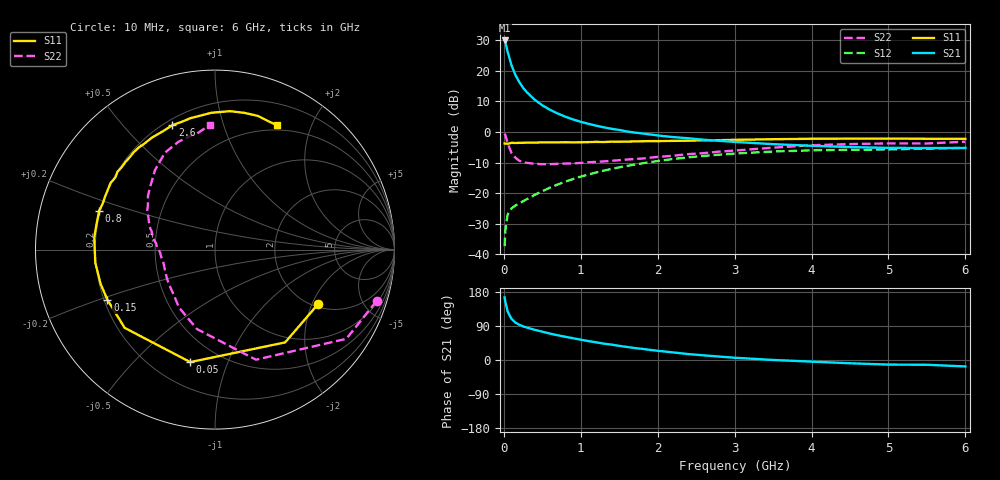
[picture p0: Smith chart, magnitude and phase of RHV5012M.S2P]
! SIEMENS Small Signal Semiconductors
! BFR106
! Si NPN RF Bipolar Junction Transistor in SOT23
! VCE = 0.5 V  IC = 12 mA
! Common Emitter S-Parameters:  August  1996
# GHz  S  MA  R  50
!  f  S11  S21  S12  S22
! GHz  MAG  ANG  MAG  ANG  MAG  ANG  MAG  ANG
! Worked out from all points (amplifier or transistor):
!   36 points, 10 MHz to 6 GHz, reference 50 ohm
!   highest |S21| = 30.0 dB at 10 MHz (marker M1)
!   |S21| within 3 dB of that: start of sweep to 42.46 MHz
!   unconditionally stable (mu >= 1): 392.1 MHz to end of sweep
!   at 250 MHz: K = 0.81, MSG = 18.6 dB, |S12| = -22.7 dB
!   at 1.4 GHz: K = 1.13, MAG = 4.4 dB, |S12| = -12.1 dB
!   at 6 GHz: K = 1.03, MAG = -1.1 dB, |S12| = -5.2 dB
!   S11 on the Smith chart (normalised r, x): 10 MHz: 2.10, -2.21; 50 MHz: 0.35, -0.74; 150 MHz: 0.21, -0.21; 800 MHz: 0.19, +0.16; 2.6 GHz: 0.23, +0.69; 6 GHz: 0.44, +1.53
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0.01  0.649 -28.1  31.61 165.1  0.0135 78.8  0.9447 -17.7
0.02  0.6482 -52.9  29.22 153.1  0.0248 67.7  0.8844 -34.2
0.05  0.6417 -102.4  20.46 127.4  0.0449 47.9  0.6545 -69.6
0.1  0.6659 -139.1  12.39 108.4  0.0561 38.8  0.4539 -102.8
0.15  0.6614 -154.9  8.615 98.9  0.0625 37.9  0.3797 -121.9
0.2  0.6655 -163.4  6.598 93.1  0.0678 39.7  0.3386 -133.4
0.25  0.6661 -169.4  5.305 88.7  0.0736 42.2  0.3209 -143.1
0.3  0.6709 -173.7  4.461 85.5  0.0794 44.8  0.3127 -148.8
0.4  0.6705 179.3  3.393 79.8  0.0931 48.7  0.3015 -157.7
0.5  0.6761 174.1  2.74 74.7  0.1074 51.4  0.297 -163.6
0.6  0.6747 169.2  2.31 69.7  0.1228 53.0  0.2976 -167.7
0.7  0.6765 165.0  2.01 65.2  0.1381 54.0  0.3013 -171.0
0.8  0.681 161.7  1.78 61.3  0.1537 54.1  0.3044 -174.3
1.1  0.6838 150.7  1.362 49.9  0.2018 53.0  0.3192 178.8
1.3  0.6851 144.1  1.193 43.2  0.2334 50.9  0.3303 174.0
1.6  0.6977 135.6  1.021 34.4  0.2788 47.3  0.354 168.0
2.2  0.7162 119.3  0.826 20.0  0.3611 38.2  0.4083 155.0
2.6  0.7328 108.9  0.747 12.2  0.4064 31.6  0.4508 146.0
3.5  0.7626 91.5  0.633 0.1  0.4795 17.2  0.5546 127.1
4.5  0.7792 77.8  0.567 -8.6  0.5115 3.2  0.6344 108.7
5.5  0.7745 67.4  0.547 -12.6  0.5348 -5.0  0.6493 99.7
6  0.7744 63.4  0.548 -17.0  0.5498 -11.2  0.6941 92.5
